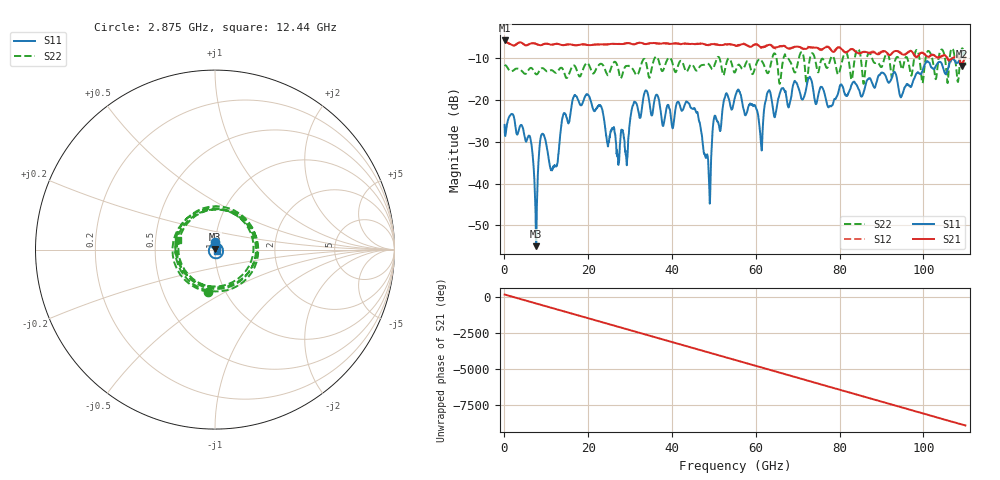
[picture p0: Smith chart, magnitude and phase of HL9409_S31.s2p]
! Created Fri Apr  1 14:40:47 2022
# ghz S ri R 50
! 2 Port Network Data from SP2.SP block
! freq  reS11  imS11  reS21  imS21  reS12  imS12  reS22  imS22
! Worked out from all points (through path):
!   2000 points, 70 MHz to 110 GHz, reference 50 ohm
!   highest |S21| = -5.73 dB at 70 MHz (marker M1); lowest = -11.9 dB at 109.1 GHz (marker M2)
!   lowest |S11| = -55.0 dB at 7.604 GHz (marker M3), VSWR 1.00, Z = 50 + j0.174 ohm
!   |S11| at or under -10 dB: start of sweep to 106.8 GHz; 106.9 GHz to 108.7 GHz (1.888 GHz wide, 1.75 % of centre)
!   |S22| runs from -16.3 to -7.6 dB; largest |S21 - S12| = 0.029
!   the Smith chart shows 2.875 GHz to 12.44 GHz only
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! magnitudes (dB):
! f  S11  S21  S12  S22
! 70 MHz  -25.9  -5.7  -5.7  -11.6
! 6.064 GHz  -28.6  -6.5  -6.6  -12.4
! 7.604 GHz  -55.0  -6.6  -6.6  -13.8
! 8.979 GHz  -28.1  -6.8  -6.8  -12.3
! 11.89 GHz  -35.9  -6.6  -6.6  -13.3
! 14.15 GHz  -23.3  -6.8  -6.8  -13.1
! 18.44 GHz  -21.2  -6.7  -6.6  -13.6
! 27.13 GHz  -34.1  -6.6  -6.6  -12.4
! 29.27 GHz  -34.8  -6.4  -6.3  -11.8
! 30.98 GHz  -20.4  -6.6  -6.6  -13.1
! 36.75 GHz  -19.4  -6.5  -6.4  -10.3
! 45.66 GHz  -22.6  -6.6  -6.5  -12.8
! 48.79 GHz  -38.3  -6.7  -6.9  -11.4
! 50.22 GHz  -23.9  -6.6  -6.6  -11.4
! 55.06 GHz  -19.2  -6.9  -6.9  -13.3
! 61.22 GHz  -30.2  -7.4  -7.3  -10.3
! 62.98 GHz  -17.9  -6.8  -6.8  -13.5
! 73.37 GHz  -15.6  -7.4  -7.5  -8.8
! 77.66 GHz  -21.4  -7.6  -7.7  -10.7
! 91.69 GHz  -15.8  -9.1  -9.2  -9.4
! 109.1 GHz  -9.4  -11.9  -11.2  -7.8
! 110 GHz  -8.6  -9.7  -9.6  -11.7
